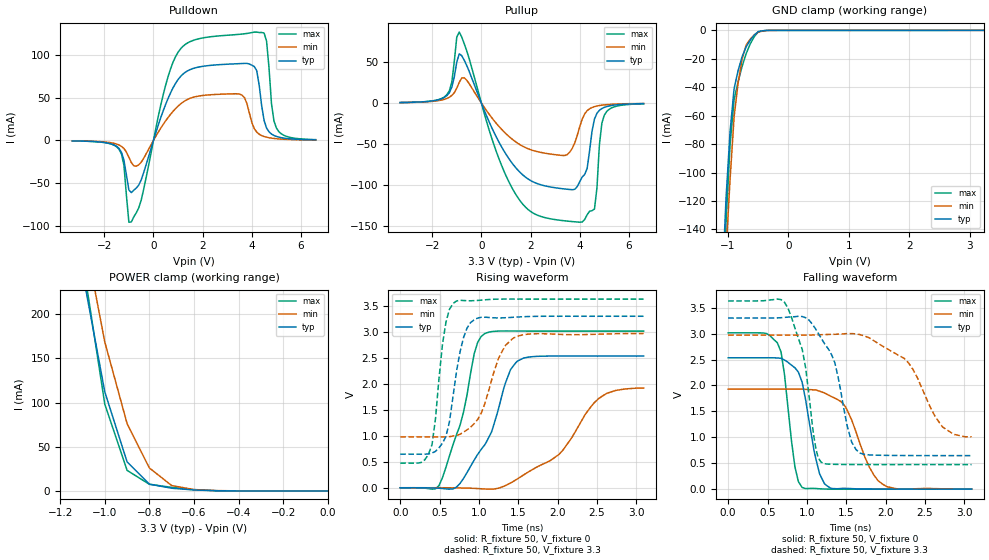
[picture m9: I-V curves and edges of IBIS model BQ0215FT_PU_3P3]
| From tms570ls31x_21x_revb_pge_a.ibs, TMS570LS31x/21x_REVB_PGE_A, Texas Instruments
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|   Model Cell BQ0215FT_PU_3P3
|BQ0215FT_PU_3P3
[Model]   BQ0215FT_PU_3P3
Model_type   I/O
Polarity   Non-Inverting
Enable   Active-Low
Vinl =  1.15
Vinh =  1.55
Cref =  15.0001pF
Rref =  101.0000M
Vref =  0V
Vmeas =  1.65
C_comp   1.2p   1.2p   1.2p
[Model Spec]
Vinl   1.15   1.02   1.28
Vinh   1.55   1.45   1.65
[Temperature Range]   25   155   -40
[Voltage Range]   3.3   2.97   3.63
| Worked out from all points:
|   slope of the pulldown table from 0 to 0.495 V, typ, clamps not added: 11.7 ohm
|   slope of the pullup table from 0 to 0.495 V, typ, clamps not added: 14.3 ohm
|   GND clamp passes 1 mA (typ) near -0.50 V on its own axis
|   POWER clamp passes 1 mA (typ) near -0.59 V on its own axis
|   rising waveform, R_fixture 50, V_fixture 0: 20-80 % time 410ps typ, 692ps min, 296ps max; typ from 0 V to 2.53 V
|   rising waveform, R_fixture 50, V_fixture 3.3: 20-80 % time 174ps typ, 268ps min, 133ps max; typ from 0.647 V to 3.3 V
|   falling waveform, R_fixture 50, V_fixture 0: 20-80 % time 182ps typ, 303ps min, 138ps max; typ from 2.53 V to 0 V
|   falling waveform, R_fixture 50, V_fixture 3.3: 20-80 % time 278ps typ, 461ps min, 209ps max; typ from 3.3 V to 0.647 V
[POWER_clamp]
|   voltage   I(typ)   I(min)   I(max)
-3.3V     4.034A     4.621A     4.844A
-1.1V     248.3mA    300.9mA    262.9mA
-1.067V   202.9mA    256.8mA    208mA
-1.033V   157.5mA    212.7mA    153.2mA
-1V       112.1mA    168.6mA    98.33mA
-900mV    32.89mA    76.22mA    23.24mA
-800mV    7.72mA     25.95mA    7.498mA
-700mV    3.046mA    6.045mA    4.01mA
-600mV    1.099mA    1.535mA    1.442mA
-500mV    196.6uA    374.7uA    217.1uA
0V        578.7pA    13.17nA    479pA
[Pulldown]
|   voltage   I(typ)   I(min)   I(max)
-3.3V     -583.8uA   -509.7uA   -562.9uA
-1.4V     -9.427mA   -5.344mA   -10.39mA
-1.2V     -23.28mA   -9.543mA   -29.38mA
-1V       -58.07mA   -19.65mA   -95.88mA
-900mV    -61.21mA   -25.99mA   -95.6mA
1V        71.34mA    40.23mA    103.4mA
3.5V      90.06mA    54.34mA    124.5mA
4.2V      81.77mA    9.741mA    127mA
4.6V      14.51mA    3.766mA    116.4mA
4.8V      7.515mA    2.688mA    43.16mA
5V        4.703mA    2.013mA    14.54mA
6.6V      667.2uA    491.6uA    918.8uA
[Pullup]
|   voltage   I(typ)   I(min)   I(max)
-3.3V     645.2uA    598.5uA    584.2uA
-1.4V     9.107mA    5.632mA    10.27mA
-900mV    59.97mA    25.19mA    86.39mA
600mV     -40.93mA   -24.45mA   -58.47mA
1.4V      -78.76mA   -47.33mA   -111.2mA
3.4V      -104.6mA   -63.8mA    -143.4mA
4V        -95.69mA   -28.77mA   -145mA
4.3V      -79.78mA   -9.339mA   -136mA
4.6V      -19.38mA   -4.395mA   -129mA
4.8V      -8.841mA   -3.032mA   -50.9mA
5V        -5.243mA   -2.22mA    -14.75mA
6.6V      -699.3uA   -541.6uA   -880.5uA
[GND_clamp]
|   voltage   I(typ)   I(min)   I(max)
-3.3V     -3.232A    -2.867A    -4.906A
-1.1V     -181.4mA   -214mA     -212mA
-1.033V   -118mA     -155.8mA   -134.9mA
-966.7mV  -71.19mA   -104.7mA   -80.42mA
-900mV    -41mA      -60.83mA   -48.65mA
-833.3mV  -28.24mA   -36.87mA   -36.03mA
-766.7mV  -18.43mA   -20.01mA   -25.25mA
-700mV    -11.56mA   -10.24mA   -16.34mA
-566.7mV  -3.329mA   -3.256mA   -4.47mA
-500mV    -899.6uA   -1.266mA   -1.048mA
-300mV    -21.34uA   -26.25uA   -33.71uA
3.233V    -1.13uA    7.014uA    -9.303uA
[Ramp]
| variable   typ   min   max
dV/dt_f   1.613131/0.2881169n   1.212883/0.4923676n   1.916028/0.2143355n
dV/dt_r   1.537307/0.4180174n   1.174497/0.7165969n   1.826328/0.2993538n
R_load = 50
[Rising Waveform]
R_fixture = 50
V_fixture = 0
V_fixture_min = 0
V_fixture_max = 0
|   time   V(typ)   V(min)   V(max)
0s        164.9uV    138.7uV    187.1uV
492ps     -8.987mV   552.4uV    40.28mV
716ps     14.55mV    -2.501mV   1.028V
804ps     180.1mV    -5.061mV   1.458V
940ps     534.8mV    -11.37mV   2.583V
1.072ns   823.9mV    -23.45mV   2.966V
1.488ns   2.437V     170.3mV    3.016V
2.016ns   2.534V     641mV      3.014V
2.516ns   2.534V     1.711V     3.014V
3.092ns   2.533V     1.917V     3.014V
[Rising Waveform]
R_fixture = 50
V_fixture = 3.3
V_fixture_min = 2.97
V_fixture_max = 3.63
|   time   V(typ)   V(min)   V(max)
0s        646.7mV    980.3mV    474.1mV
268ps     646.2mV    980.4mV    487.8mV
404ps     668.1mV    979.8mV    832.3mV
580ps     985.8mV    980mV      3.181V
716ps     2.248V     1.007V     3.595V
892ps     3.175V     1.165V     3.598V
1.028ns   3.28V      1.434V     3.61V
1.248ns   3.267V     2.488V     3.629V
1.444ns   3.281V     2.885V     3.631V
3.092ns   3.3V       2.968V     3.63V
[Falling Waveform]
R_fixture = 50
V_fixture = 0
V_fixture_min = 0
V_fixture_max = 0
|   time   V(typ)   V(min)   V(max)
0s        2.534V     1.93V      3.014V
624ps     2.53V      1.93V      2.826V
716ps     2.49V      1.93V      2.206V
848ps     2.341V     1.931V     431mV
940ps     2.061V     1.929V     32.56mV
1.16ns    303mV      1.889V     7.652mV
1.292ns   28.09mV    1.8V       1.137mV
1.488ns   15.02mV    1.593V     410.2uV
1.96ns    695.7uV    98.62mV    419.5uV
3.092ns   444.3uV    1.597mV    218.8uV
[Falling Waveform]
R_fixture = 50
V_fixture = 3.3
V_fixture_min = 2.97
V_fixture_max = 3.63
|   time   V(typ)   V(min)   V(max)
0s        3.3V       2.97V      3.63V
760ps     3.318V     2.97V      3.489V
940ps     3.329V     2.97V      2.701V
1.092ns   3.132V     2.973V     982.4mV
1.18ns    2.916V     2.978V     522.2mV
1.356ns   2.433V     2.987V     478.7mV
1.68ns    692.7mV    2.978V     474.5mV
2.292ns   648.2mV    2.433V     474.3mV
2.724ns   646.7mV    1.198V     474.2mV
3.092ns   646.6mV    1.01V      474.2mV
